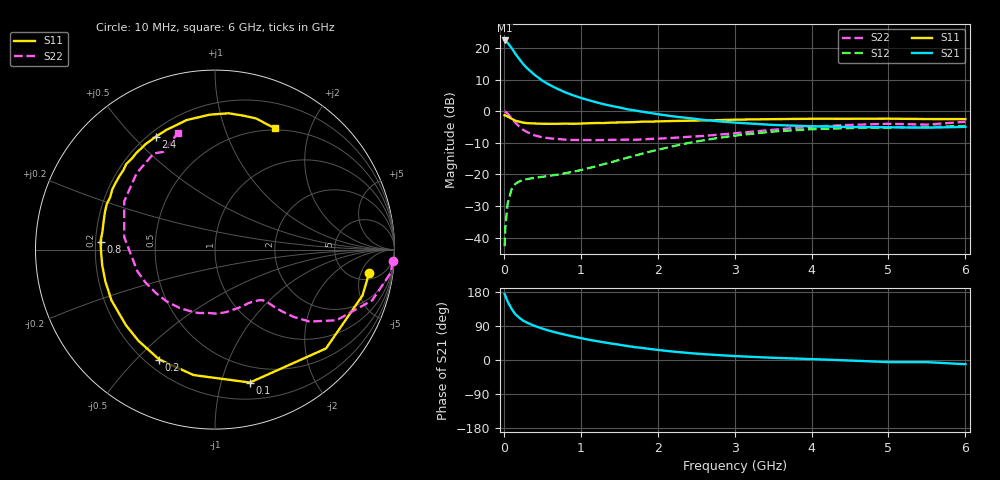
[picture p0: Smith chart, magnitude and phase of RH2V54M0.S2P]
! SIEMENS Small Signal Semiconductors
! BFR106
! Si NPN RF Bipolar Junction Transistor in SOT23
! VCE = 2.5 V  IC = 4 mA
! Common Emitter S-Parameters:  August  1996
# GHz  S  MA  R  50
!  f  S11  S21  S12  S22
! GHz  MAG  ANG  MAG  ANG  MAG  ANG  MAG  ANG
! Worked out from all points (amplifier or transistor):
!   36 points, 10 MHz to 6 GHz, reference 50 ohm
!   highest |S21| = 22.5 dB at 10 MHz (marker M1)
!   |S21| within 3 dB of that: start of sweep to 117.3 MHz
!   unconditionally stable (mu >= 1): 658.1 MHz to 2.088 GHz; 4.183 GHz to end of sweep
!   at 250 MHz: K = 0.45, MSG = 18.4 dB, |S12| = -21.7 dB
!   at 1.4 GHz: K = 1.18, MAG = 6.3 dB, |S12| = -16.1 dB
!   at 6 GHz: K = 1.02, MAG = -1.1 dB, |S12| = -4.6 dB
!   S11 on the Smith chart (normalised r, x): 10 MHz: 6.59, -7.06; 100 MHz: 0.35, -1.24; 200 MHz: 0.25, -0.59; 800 MHz: 0.22, +0.03; 2.4 GHz: 0.23, +0.58; 6 GHz: 0.48, +1.51
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0.01  0.8687 -8.7  13.29 174.0  0.0073 88.0  0.9938 -3.8
0.02  0.8606 -17.3  13.1 169.4  0.0147 80.7  0.9862 -7.7
0.05  0.8281 -41.7  12.16 154.0  0.035 68.6  0.9201 -17.9
0.1  0.7657 -75.3  10.14 135.3  0.0579 53.8  0.7831 -30.2
0.15  0.7091 -99.7  8.177 120.8  0.0709 43.8  0.6615 -37.3
0.2  0.6866 -116.9  6.782 111.6  0.0773 38.8  0.5754 -40.6
0.25  0.6632 -130.1  5.66 104.0  0.0819 35.5  0.5101 -42.6
0.3  0.6509 -139.7  4.853 98.6  0.0843 34.5  0.4715 -43.7
0.4  0.6424 -153.9  3.79 90.0  0.0884 33.6  0.4165 -45.1
0.5  0.6361 -163.8  3.073 82.9  0.0918 34.8  0.3874 -46.7
0.6  0.6344 -172.1  2.606 76.7  0.0955 37.2  0.3735 -49.1
0.8  0.6394 176.0  1.999 66.6  0.1047 42.9  0.3561 -55.2
1.1  0.6477 161.3  1.506 53.7  0.1258 51.7  0.3501 -66.8
1.3  0.653 153.3  1.297 46.6  0.1457 55.7  0.3503 -75.3
1.6  0.6712 142.7  1.081 37.0  0.1837 59.1  0.3564 -89.7
2.2  0.7033 123.6  0.833 22.2  0.2803 56.5  0.3801 -121.1
2.4  0.7101 117.7  0.782 18.5  0.3151 53.8  0.3947 -132.9
3.5  0.7524 92.2  0.609 5.8  0.4787 33.0  0.5103 172.2
4.5  0.7629 77.9  0.566 -1.4  0.5431 13.8  0.6097 135.7
5  0.7658 72.5  0.559 -5.5  0.5557 6.3  0.6352 122.5
5.5  0.7553 67.0  0.551 -5.6  0.5634 2.6  0.6165 118.0
6  0.7546 63.5  0.568 -11.1  0.5873 -5.0  0.6837 107.4
